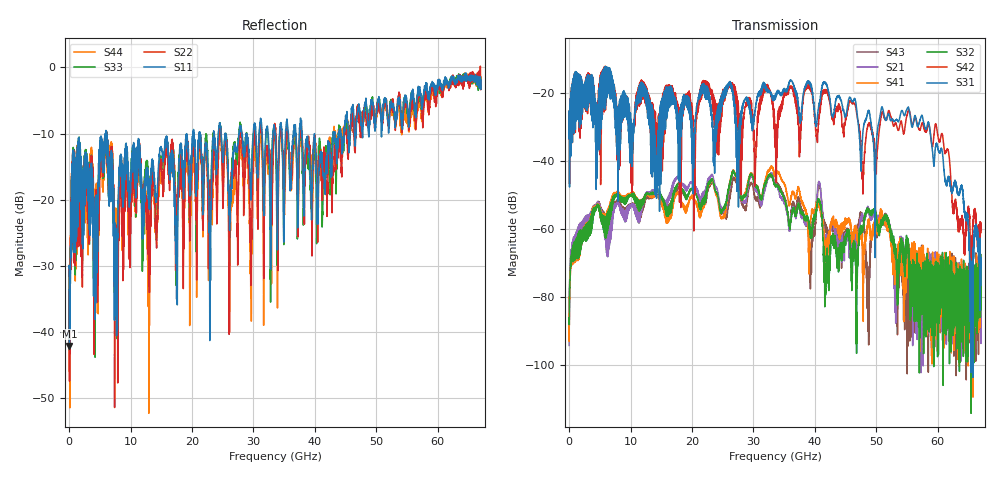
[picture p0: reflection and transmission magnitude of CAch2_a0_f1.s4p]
!Agilent Technologies,N5247A,US51170199,A.09.90.13
!Agilent N5247A: A.09.90.13
!Date: Thursday, October 18, 2018 12:05:38
!Correction: S11(Full 4 Port(1,2,3,4))
!S12(Full 4 Port(1,2,3,4))
!S13(Full 4 Port(1,2,3,4))
!S14(Full 4 Port(1,2,3,4))
!S21(Full 4 Port(1,2,3,4))
!S22(Full 4 Port(1,2,3,4))
!S23(Full 4 Port(1,2,3,4))
!S24(Full 4 Port(1,2,3,4))
!S31(Full 4 Port(1,2,3,4))
!S32(Full 4 Port(1,2,3,4))
!S33(Full 4 Port(1,2,3,4))
!S34(Full 4 Port(1,2,3,4))
!S41(Full 4 Port(1,2,3,4))
!S42(Full 4 Port(1,2,3,4))
!S43(Full 4 Port(1,2,3,4))
!S44(Full 4 Port(1,2,3,4))
!S4P File: Measurements: <S11,S12,S13,S14>,
!<S21,S22,S23,S24>,
!<S31,S32,S33,S34>,
!<S41,S42,S43,S44>:
# Hz S  dB  R 50
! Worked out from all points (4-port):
!   6701 points, 10 MHz to 67 GHz, reference 50 ohm
!   strongest paths, dB at 10 MHz, 16.76 GHz, 33.51 GHz, 50.25 GHz, 67 GHz:
!     S31: -33.3, -23.0, -21.0, -29.9, -76.7
!     S42: -33.4, -18.5, -29.5, -35.0, -60.3
!     S32: -86.1, -51.5, -47.0, -59.5, -82.4
!     S41: -85.0, -53.5, -44.4, -59.9, -73.4
!     S21: -94.3, -47.6, -46.2, -57.1, -75.7
!     S43: -85.3, -51.5, -47.3, -59.8, -80.2
!   lowest |S11| = -42.1 dB at 69.99 MHz (marker M1), VSWR 1.02, Z = 50.2 + j0.763 ohm
!   |S11| at or under -10 dB: start of sweep to 5.894 GHz; 6.106 GHz to 20.16 GHz (14.05 GHz wide, 107 % of centre); 37.92 GHz to 43 GHz (5.078 GHz wide, 12.6 % of centre)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
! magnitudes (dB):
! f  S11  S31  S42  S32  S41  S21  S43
! 10 MHz  -30.3  -33.3  -33.4  -86.1  -85.0  -94.3  -85.3
! 69.99 MHz  -42.1  -32.8  -32.5  -81.1  -80.1  -79.4  -78.7
! 7.699 GHz  -25.7  -23.6  -23.5  -49.7  -49.1  -52.4  -51.8
! 32.78 GHz  -26.7  -19.6  -20.1  -43.9  -41.8  -43.7  -44.0
! 41.91 GHz  -16.1  -17.8  -19.2  -68.6  -64.5  -63.7  -60.6
! 55.1 GHz  -6.5  -24.2  -25.7  -65.1  -67.6  -66.4  -77.3
! 67 GHz  -3.3  -76.7  -60.3  -82.4  -73.4  -75.7  -80.2
